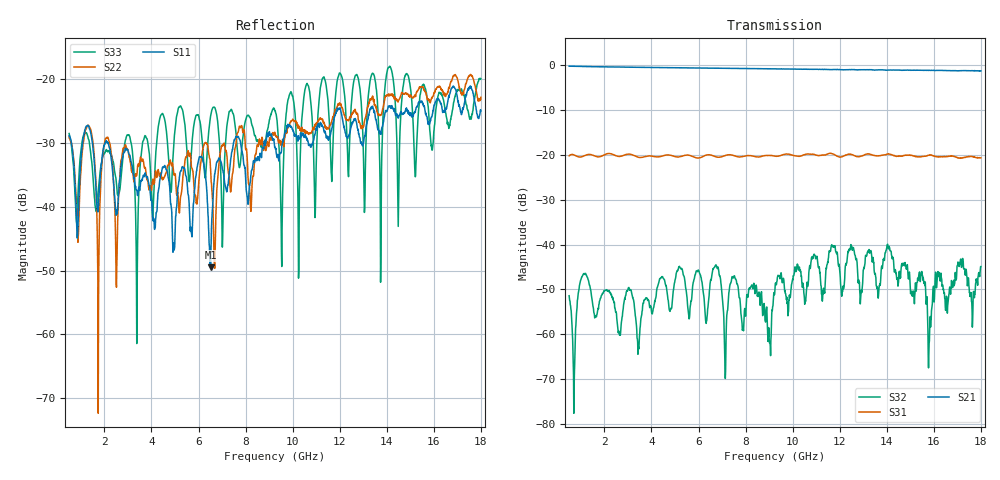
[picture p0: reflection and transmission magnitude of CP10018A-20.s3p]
! Amtery
! Email: info@amtery.com
! Phone: 886-2-2883-7839
! Model Number: CP10018A-20
! 3-port S-parameter measurement data for Directional Coupler
! Frequency Range: 0.5 GHz to 18 GHz
! Port 1: Input
! Port 2: Output
! Port 3: Coupled
# hz S db R 50
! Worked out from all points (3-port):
!   1401 points, 500 MHz to 18 GHz, reference 50 ohm
!   strongest paths, dB at 500 MHz, 4.875 GHz, 9.25 GHz, 13.62 GHz, 18 GHz:
!     S21: -0.2, -0.5, -0.8, -1.0, -1.2
!     S31: -20.2, -20.1, -20.2, -20.2, -20.6
!     S32: -51.4, -53.4, -49.9, -51.7, -44.9
!   lowest |S11| = -49.5 dB at 6.513 GHz (marker M1), VSWR 1.01, Z = 50.2 - j0.289 ohm
!   |S11| at or under -10 dB: start of sweep to end of sweep
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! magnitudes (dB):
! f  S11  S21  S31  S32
! 500 MHz  -28.9  -0.2  -20.2  -51.4
! 1.738 GHz  -40.5  -0.3  -20.4  -54.2
! 2.062 GHz  -29.8  -0.3  -19.8  -50.2
! 3.375 GHz  -37.5  -0.4  -20.4  -59.1
! 6.513 GHz  -49.5  -0.6  -20.0  -47.9
! 9.037 GHz  -28.9  -0.7  -20.1  -62.0
! 9.25 GHz  -30.7  -0.8  -20.2  -49.9
! 9.525 GHz  -31.3  -0.8  -20.0  -46.9
! 9.912 GHz  -27.5  -0.8  -19.9  -51.2
! 18 GHz  -25.1  -1.2  -20.6  -44.9
